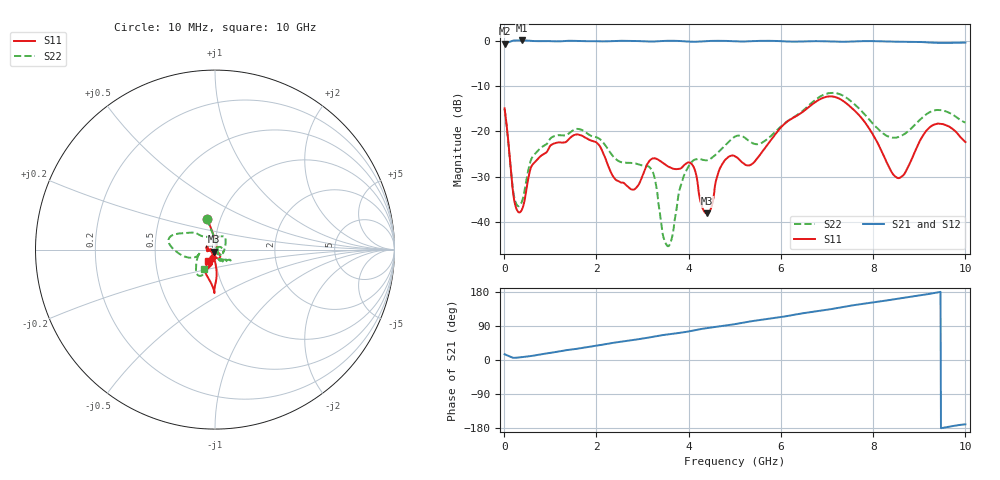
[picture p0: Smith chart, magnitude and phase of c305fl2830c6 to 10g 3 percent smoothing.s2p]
!Agilent Technologies,N5234A,MY52241123,A.10.00.00
!Agilent N5234A: A.10.00.00
!Date: Monday, May 06, 2019 15:05:17
!Correction: S11(Full 2 Port(1,2))
!S21(Full 2 Port(1,2))
!S12(Full 2 Port(1,2))
!S22(Full 2 Port(1,2))
!S2P File: Measurements: S11, S21, S12, S22:
# Hz S  dB  R 50
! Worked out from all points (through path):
!   1001 points, 10 MHz to 10 GHz, reference 50 ohm
!   highest |S21| = 0.03 dB at 379.6 MHz (marker M1); lowest = -0.7 dB at 10 MHz (marker M2)
!   lowest |S11| = -38.1 dB at 4.396 GHz (marker M3), VSWR 1.03, Z = 49.5 - j1.13 ohm
!   |S11| at or under -10 dB: start of sweep to end of sweep
!   |S22| runs from -45.4 to -11.5 dB; largest |S21 - S12| = 0.0015
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1e7  -14.95 104.8  -0.65 15.1  -0.64 15.2  -15.08 105.4
2.1979e8  -35.34 45.3  0.02 5.7  0.02 5.7  -34.64 44.4
3.7963e8  -37.43 -34.3  0.03 7.5  0.03 7.5  -35.69 -23.2
6.5935e8  -26.89 -106.3  -0.10 12.1  -0.11 12.1  -25.11 -69.1
1.67833e9  -20.94 -108.3  -0.12 31.6  -0.12 31.6  -19.69 -35.2
2.76724e9  -32.87 -149.7  -0.08 52.2  -0.08 52.2  -27.03 -52.0
3.18682e9  -26.19 170.6  -0.20 60.5  -0.20 60.5  -28.35 -48.0
3.34666e9  -26.33 159.3  -0.15 64.1  -0.15 64.0  -36.05 -53.6
3.45655e9  -27.09 160.2  -0.08 66.1  -0.08 66.0  -43.51 -8.4
3.56644e9  -27.85 166.7  -0.04 67.8  -0.04 67.8  -45.33 26.9
3.92608e9  -27.28 -167.7  -0.17 73.8  -0.17 73.8  -29.17 23.5
4.1059e9  -27.84 -176.6  -0.26 77.9  -0.26 77.9  -26.42 -10.6
4.39561e9  -38.13 -112.8  -0.11 84.2  -0.11 84.2  -26.41 -17.0
4.7053e9  -27.67 -48.1  -0.05 89.3  -0.06 89.3  -24.01 23.2
5.005e9  -25.53 -69.8  -0.15 94.6  -0.15 94.6  -21.19 49.0
5.36464e9  -27.30 -84.9  -0.13 102.4  -0.13 102.4  -22.55 76.4
6.67333e9  -14.11 -95.1  -0.12 126.9  -0.12 126.8  -13.69 153.9
7.43257e9  -13.96 -90.0  -0.24 141.7  -0.24 141.7  -12.69 179.2
8.34166e9  -27.84 -99.7  -0.21 158.1  -0.21 158.0  -21.21 -168.0
8.63137e9  -29.90 -104.0  -0.25 163.7  -0.25 163.7  -20.91 -167.2
9.34066e9  -18.48 -113.4  -0.49 177.1  -0.49 177.0  -15.39 -125.7
1e10  -22.39 -122.4  -0.45 -169.7  -0.45 -169.8  -18.11 -119.3
